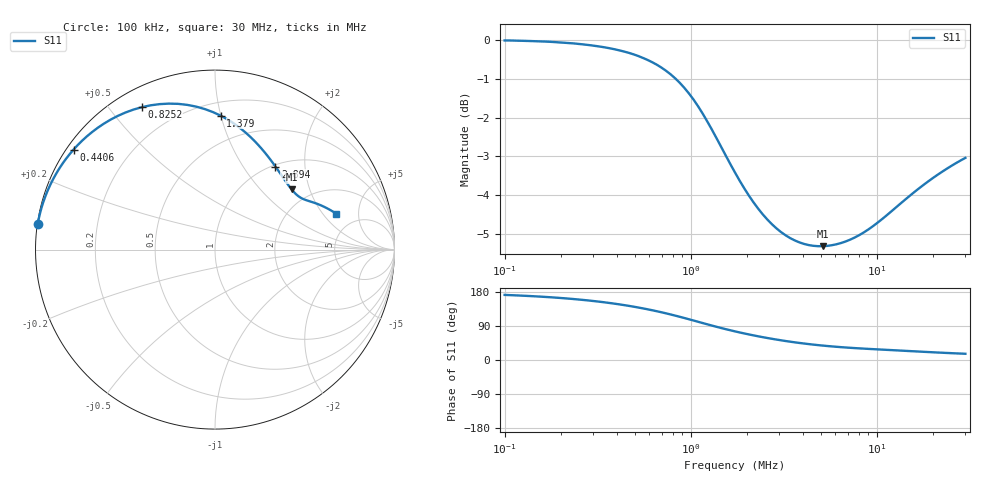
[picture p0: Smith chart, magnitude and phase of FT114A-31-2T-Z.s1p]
! ListType=Log
!!FT114A-31 2T Z
# MHz S RI R 50
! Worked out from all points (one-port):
!   101 points, 100 kHz to 30 MHz, reference 50 ohm
!   lowest |S11| = -5.3 dB at 5.119 MHz (marker M1), VSWR 3.38, Z = 80.1 + j76.1 ohm
!   |S11| at or under -10 dB: nowhere
!   S11 on the Smith chart (normalised r, x): 100 kHz: 0.00, +0.07; 440.6 kHz: 0.02, +0.32; 825.2 kHz: 0.08, +0.61; 1.379 MHz: 0.30, +1.00; 2.894 MHz: 1.03, +1.42; 30 MHz: 3.48, +2.76
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0.1  -0.9873 0.143
0.1490728  -0.9726 0.2109
0.2099064  -0.9468 0.2922
0.2637003  -0.9178 0.3607
0.3129135  -0.8866 0.42
0.3713111  -0.8445 0.486
0.4406071  -0.7882 0.5571
0.5228356  -0.714 0.6309
0.62041  -0.6184 0.7022
0.6953784  -0.5418 0.7448
0.8251537  -0.4079 0.7934
0.8735868  -0.3589 0.8039
0.9791484  -0.257 0.8133
1.097466  -0.1543 0.8063
1.23008  -0.0564 0.7829
1.378719  0.0315 0.7463
1.545319  0.1065 0.7017
1.833715  0.1954 0.6295
2.055296  0.2413 0.5828
2.303651  0.2791 0.539
2.89402  0.3371 0.4624
3.635686  0.3795 0.4011
5.119336  0.4273 0.335
7.631539  0.4754 0.2904
10.15005  0.5142 0.2734
15.13097  0.5784 0.2514
21.30561  0.6314 0.2265
30  0.6761 0.1996
